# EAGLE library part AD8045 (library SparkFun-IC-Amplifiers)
Unity-gain stable feedback amplifier Low noise, low distortion, 1GHz BW. Datasheet SparkFun Products SparkFun MiniGen - Pro Mini Signal Generator Shield (BOB-11420)
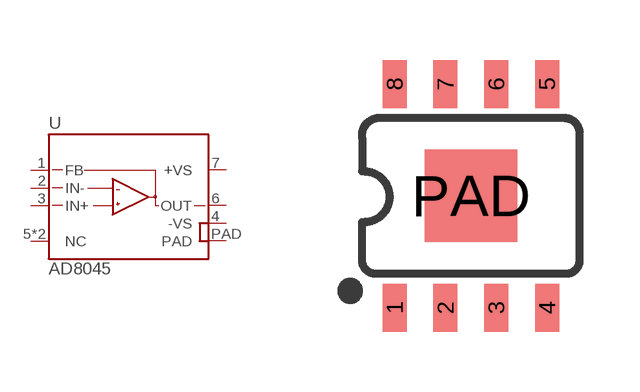
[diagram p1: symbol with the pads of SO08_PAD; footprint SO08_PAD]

Designator prefix U

## AD8045-PAD (PROD_ID: IC-11224; VALUE: ADC8045)  [SO08_PAD]
1  FB
2  IN-
3  IN+
4  -VS  pwr
5  NC  nc
6  OUT
7  +VS  pwr
8  NC  nc
PAD  PAD  pwr

## Footprint SO08_PAD (pad centres in mm)
SOIC, 0.15 inch width
smd 0.6 x 1.2: 1 -1.905,-2.8; 2 -0.635,-2.8; 3 0.635,-2.8; 4 1.905,-2.8; 5 1.905,2.8; 6 0.635,2.8; 7 -0.635,2.8; 8 -1.905,2.8
smd 2.311 x 2.311: PAD 0,0

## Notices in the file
Licensing: Creative Commons ShareAlike 4.0 International - https://creativecommons.org/licenses/by-sa/4.0
